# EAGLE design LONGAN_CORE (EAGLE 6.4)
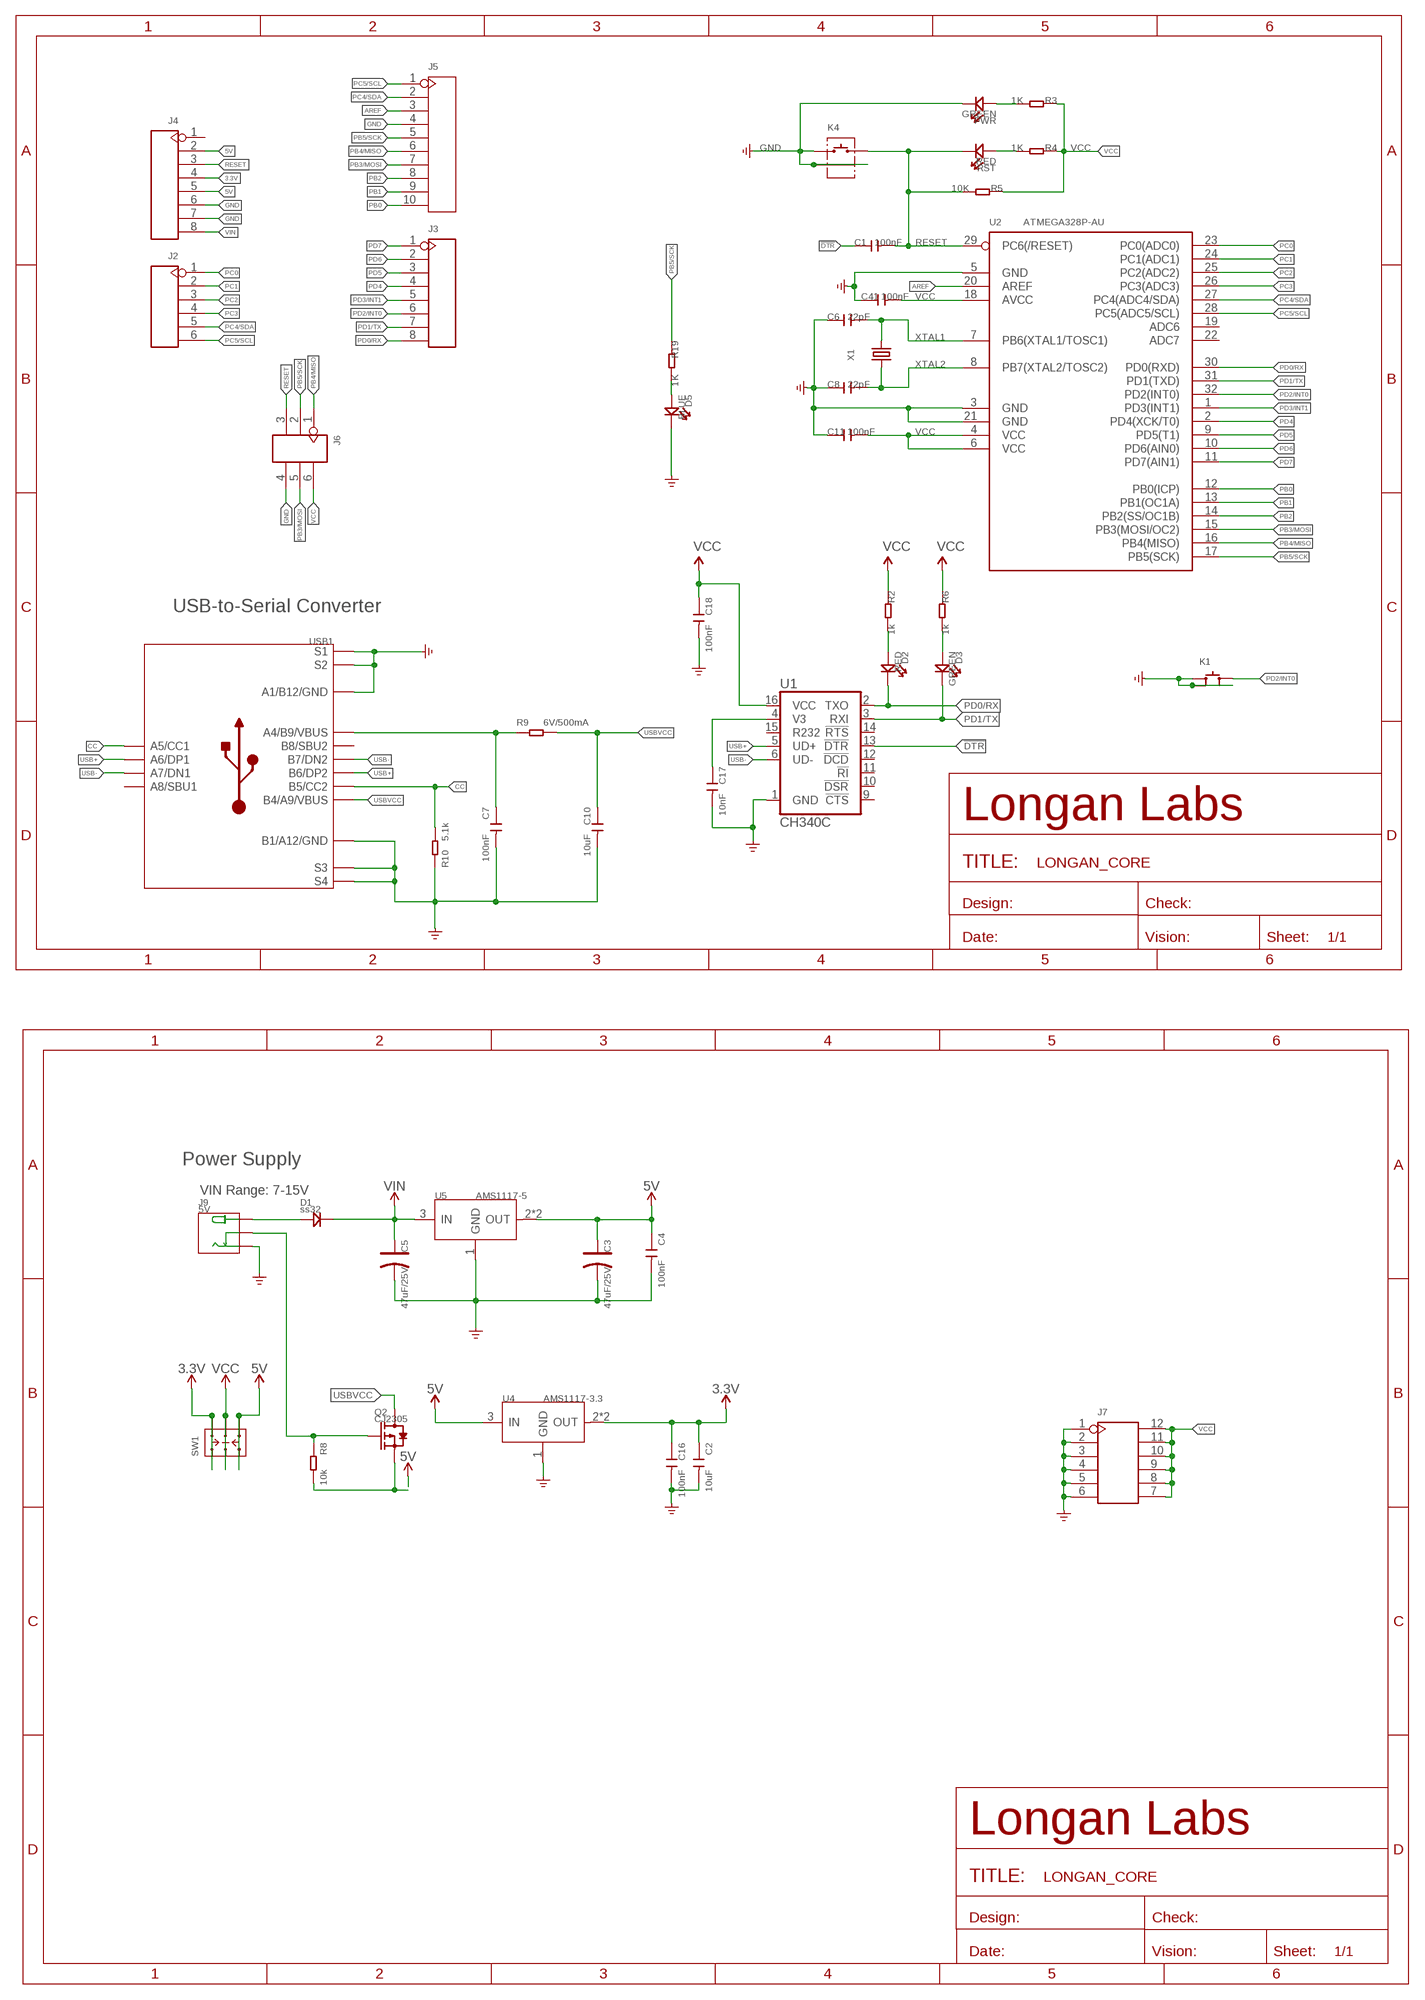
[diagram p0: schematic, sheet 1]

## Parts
C1  100nF  C-0603  [C0603]
C2  10uF  CAP-0603  [C0603]
C3  47uF/25V  CAP-POLAR-ELECTRO-C  [ELECTRO-SMD-C-6MM]
C4  100nF  CAP-0603  [C0603]
C5  47uF/25V  CAP-POLAR-ELECTRO-C  [ELECTRO-SMD-C-6MM]
C6  22pF  C-0603  [C0603]
C7  100nF  CAP-0603  [C0603]
C8  22pF  C-0603  [C0603]
C10  10uF  CAP-0603  [C0603]
C11  100nF  C-0603  [C0603]
C16  100nF  CAP-0603  [C0603]
C17  10nF  CAP-0603  [C0603]
C18  100nF  CAP-0603  [C0603]
C41  100nF  C-0603  [C0603]
D1  ss32  DIODE'SMA'  [DO-214AC]
D2  RED  LED'0603'  [LED-0603]
D3  GREEN  LED'0603'  [LED-0603]
D5  BLUE  LED'0603'  [LED-0603]
J2  HEADER-6P-55/35MIL  [H6-2.54]
J3  HEADER-8P-65/35MIL  [H8-2.54-C65D35MIL]
J4  HEADER-8P-65/35MIL  [H8-2.54-C65D35MIL]
J5  HEADER-10P-2.54  [H10-2.54]
J6  HEADER-2X3P-2.54  [H2X3-2.54]
J7  HEADER-2X6P-2.54  [H2X6-2.54]
J9  5V  POWER-JACK-DC-320120003  [DCJ3P-14.2X11.0X9.0MM]
K1  BUTTON-4P-6.2X6.2  [SW4-SMD-6.2X6.2MM]
K4  BUTTON-2+2P  [SW2+2P-7.7X2.75X3.95MM]
PWR  GREEN  LED'0603'  [LED-0603]
Q2  CJ2305  MOSFET-P'SI2323CDS/SI2305DS<BR>'  [SOT-23]
R2  1k  R-0603  [R0603]
R3  1K  R-0603  [R0603]
R4  1K  R-0603  [R0603]
R5  10K  R-0603  [R0603]
R6  1k  R-0603  [R0603]
R8  10k  RES-0603  [R0603]
R9  6V/500mA  RES-0805  [R0805]
R10  5.1k  RES-0603  [R0603]
R19  1K  R-0603  [R0603]
RST  RED  LED'0603'  [LED-0603]
SW1  SWITCH-2CH-6P-311010004  [SW6-2.54-9.0X3.5X3.2+2.0MM]
U1  CH340C  [SO016]
U2  ATMEGA328P-AU  MCU-ATMEGA8/168/328'AU'  [TQFP32-0.8-7X7MM]
U4  AMS1117-3.3  PMIC-CJ1117S  [SOT-223]
U5  AMS1117-5  PMIC-CJ1117S  [SOT-223]
USB1  TYPE-C-31-M-12  USB2.0-TYPE-C  [USB2.0-TYPE-C]
X1  16MHz  CRYSTAL-2P'HC49US'  [HC49US]

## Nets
3.3V: C2.1 C16.1 J4.4 SW1.CH1A SW1.CH2A U4.2(OUT) U4.TER(OUT)
5V: C3.+ C4.1 J4.2 J4.5 Q2.2(S) R8.2 SW1.CH1B SW1.CH2B U4.3(IN) U5.2(OUT) U5.TER(OUT)
!DTR: C1.1 U1.13(!DTR)
AREF: J5.3 U2.20(AREF)
CC: R10.2 USB1.A5(A5/CC1) USB1.B5(B5/CC2)
GND: C2.2 C3.- C4.2 C5.- C6.1 C7.2 C8.1 C10.2 C11.1 C16.2 C17.2 C18.2 C41.1 D5.- J4.6 J4.7 J5.4 J6.4 J7.1 J7.2 J7.3 J7.4 J7.5 J7.6 J9.-1(-) K1.1(A0) K1.3(B1) K1.4(A1) K4.1 K4.S1 K4.S2 PWR.- R10.1 U1.1(GND) U2.3(GND) U2.5(GND) U2.21(GND) U4.1(GND) U5.1(GND) USB1.A1_B12(A1/B12/GND) USB1.B1_A12(B1/A12/GND) USB1.S1 USB1.S2 USB1.S3 USB1.S4 USB1.S5(S1) USB1.S6(S2) ; supply symbol labelled GND_POWER
INSERT: J9.-2(CDN) Q2.1(G) R8.1
N$3: D5.+ R19.2
N$4: C7.1 R9.1 USB1.A4_B9(A4/B9/VBUS)
N$5: D3.+ R6.2
N$6: C17.1 U1.4(V3)
N$7: PWR.+ R3.2
N$9: D2.+ R2.2
N$17: R4.2 RST.+
PB0: J5.10 U2.12(PB0(ICP))
PB1: J5.9 U2.13(PB1(OC1A))
PB2: J5.8 U2.14(PB2(SS/OC1B))
PB3/MOSI: J5.7 J6.5 U2.15(PB3(MOSI/OC2))
PB4/MISO: J5.6 J6.1 U2.16(PB4(MISO))
PB5/SCK: J5.5 J6.2 R19.1 U2.17(PB5(SCK))
PC0: J2.1 U2.23(PC0(ADC0))
PC1: J2.2 U2.24(PC1(ADC1))
PC2: J2.3 U2.25(PC2(ADC2))
PC3: J2.4 U2.26(PC3(ADC3))
PC4/SDA: J2.5 J5.2 U2.27(PC4(ADC4/SDA))
PC5/SCL: J2.6 J5.1 U2.28(PC5(ADC5/SCL))
PD0/RX: D2.- J3.8 U1.2(TXO) U2.30(PD0(RXD))
PD1/TX: D3.- J3.7 U1.3(RXI) U2.31(PD1(TXD))
PD2/INT0: J3.6 K1.2(B0) U2.32(PD2(INT0))
PD3/INT1: J3.5 U2.1(PD3(INT1))
PD4: J3.4 U2.2(PD4(XCK/T0))
PD5: J3.3 U2.9(PD5(T1))
PD6: J3.2 U2.10(PD6(AIN0))
PD7: J3.1 U2.11(PD7(AIN1))
PWRIN: D1.1(+) J9.+
RESET: C1.2 J4.3 J6.3 K4.2 R5.2 RST.- U2.29(PC6(/RESET))
USB+: U1.5(UD+) USB1.A6(A6/DP1) USB1.B6(B6/DP2)
USB-: U1.6(UD-) USB1.A7(A7/DN1) USB1.B7(B7/DN2)
USBVCC: C10.1 Q2.3(D) R9.2 USB1.B4_A9(B4/A9/VBUS)
VCC: C11.2 C18.1 C41.2 J6.6 J7.7 J7.8 J7.9 J7.10 J7.11 J7.12 R2.1 R3.1 R4.1 R5.1 R6.1 SW1.COM1 SW1.COM2 U1.16(VCC) U2.4(VCC) U2.6(VCC) U2.18(AVCC)
VIN: C5.+ D1.2(-) J4.8 U5.3(IN)
XTAL1: C6.2 U2.7(PB6(XTAL1/TOSC1)) X1.2
XTAL2: C8.2 U2.8(PB7(XTAL2/TOSC2)) X1.1
Unconnected: J4.1 U1.9(!CTS) U1.10(!DSR) U1.11(!RI) U1.12(!DCD) U1.14(!RTS) U1.15(R232) U2.19(ADC6) U2.22(ADC7) USB1.A8(A8/SBU1) USB1.B8(B8/SBU2)

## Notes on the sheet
- USB-to-Serial Converter
- Power Supply
- VIN Range: 7-15V

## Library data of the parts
C1 C6 C8 C11 C41 = Discrete:C*: Ceramic Capacitors
C2 C4 C7 C10 C16-C18 = Discrete-new:CAP: Ceramic Capacitors
C3 C5 = Discrete-new:CAP-POLAR: Electrolytic Capacitors,Tantalum Capacitors and Super Capacitors
D1 = Discrete-new:DIODE
D2 D3 D5 PWR RST = Discrete-new:LED
J2 = Connector-new:HEADER-6P
J3 J4 = Connector-new:HEADER-8P
J5 = Connector-new:HEADER-10P
J6 = Connector-new:HEADER-2X3P
J7 = Connector-new:HEADER-2X6P
J9 = Connector-new:POWER-JACK-DC
K1 = Switch:BUTTON-4P
K4 = Connector-new:BUTTON-2+2P
Q2 = Discrete-new:MOSFET-P
R2-R6 R19 = Discrete:R*
R8-R10 = Discrete-new:RES
SW1 = Switch:SWITCH-2CH-6P
U1 = SparkFun-IC-Comms:CH340C; PROD_ID: IC-14038
U2 = IC-new:MCU-ATMEGA8/168/328
U4 U5 = IC-new:PMIC-CJ*1117: Low Drop Fixed And Adjustable Positive Voltage Regulators http://www.datasheetcatalog.org/datasheet/SGSThomsonMicroelectronics/mXuqtqv.pdf
USB1 = Connector-new:USB2.0-TYPE-C
X1 = Discrete-new:CRYSTAL-2P

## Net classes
1 power: width 0.152 mm, drill 0.152 mm, clearance 0.152 mm
2 gnd: width 0.152 mm, drill 0.152 mm, clearance 0.152 mm
3 usbvcc: width 0.152 mm, drill 0.152 mm, clearance 0.152 mm

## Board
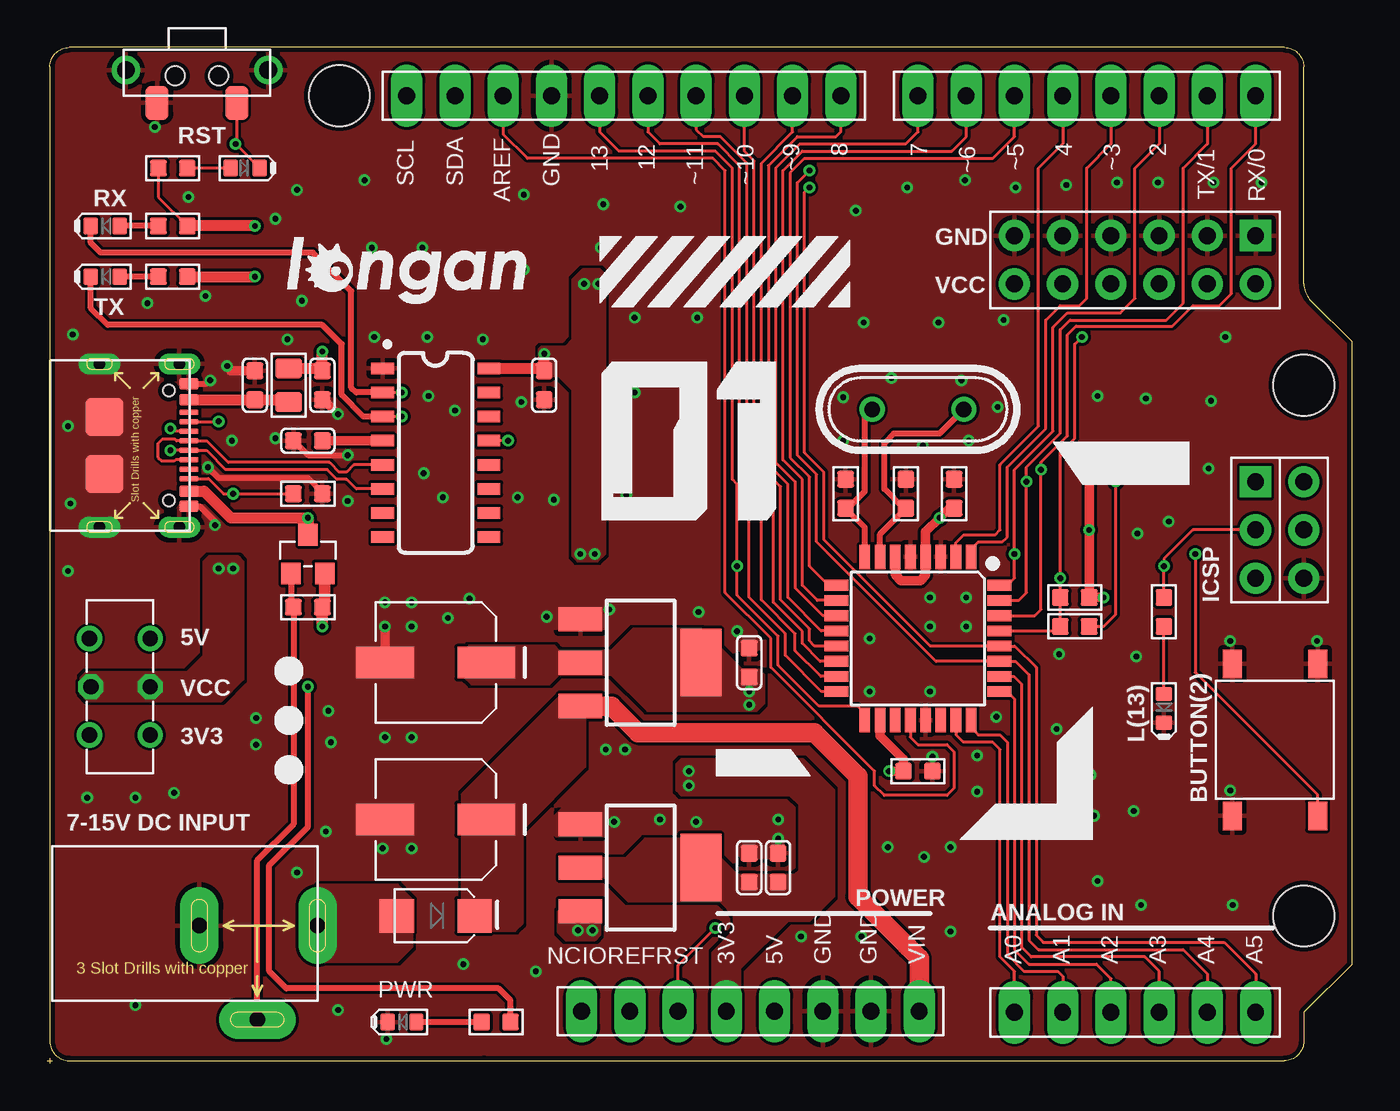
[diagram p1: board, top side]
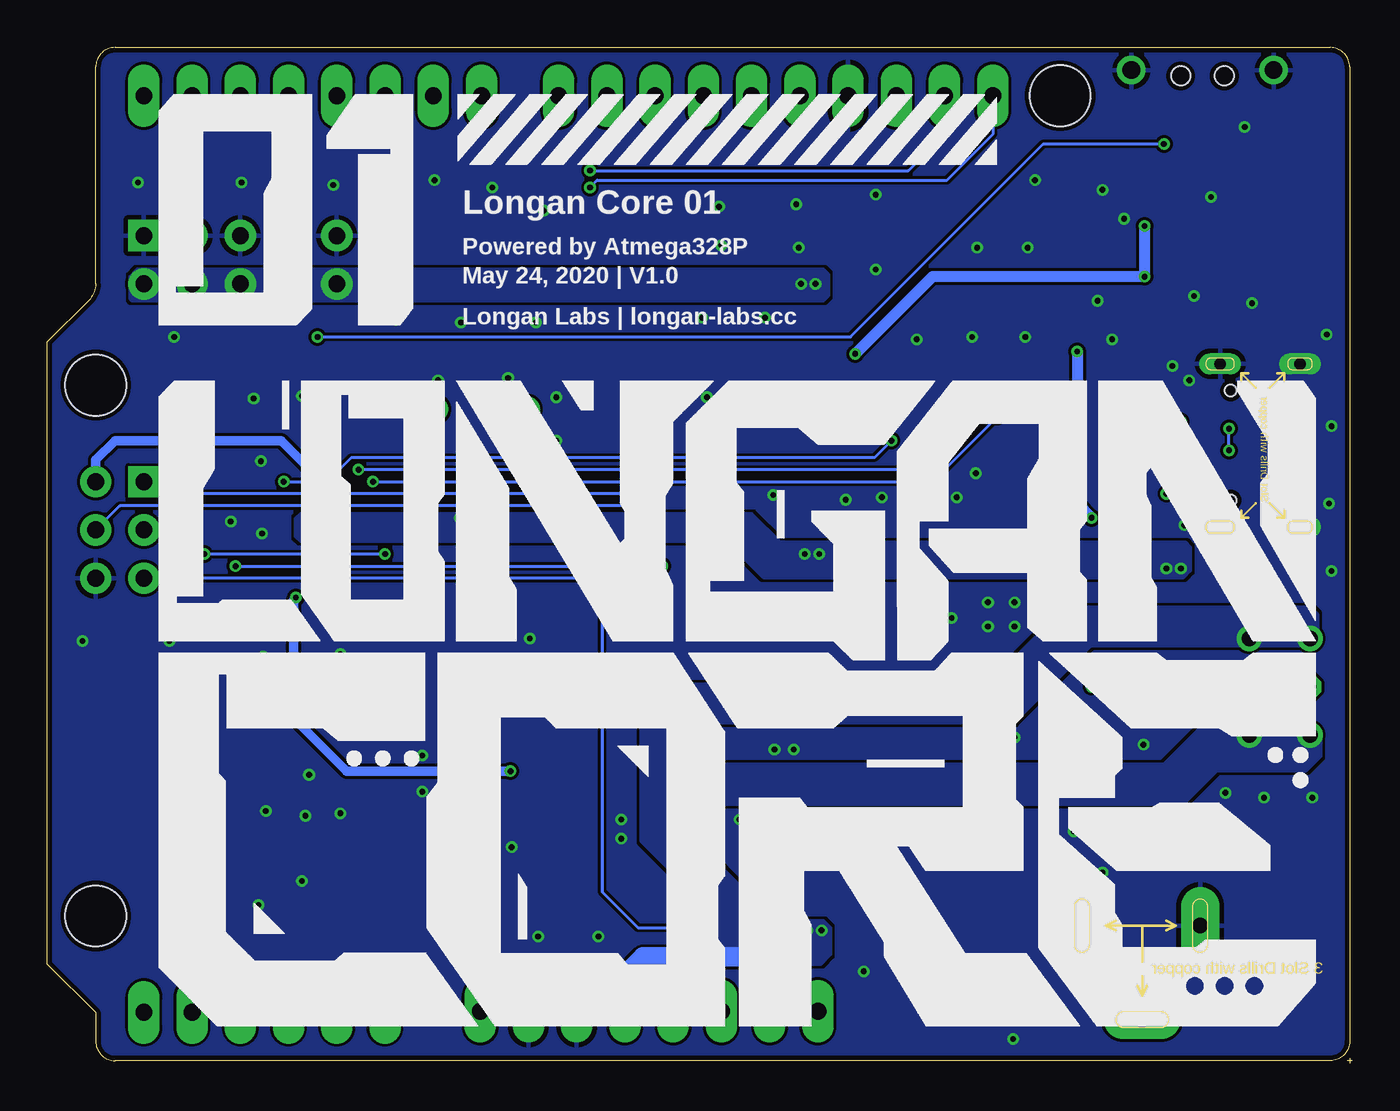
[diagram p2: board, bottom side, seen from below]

Size 68.71 x 53.47 mm. Coordinates in mm from the lower left corner, seen from the top.
Outline: 66.17,41.04 arc45 66.54,40.14 68.71,37.97 68.71,5.21 66.17,2.67 66.17,1.14 arc-90 65.15,0.13 23,0.13
Outline: 66.17,41.02 66.17,52.45 arc90 65.15,53.47 1.14,53.47 arc90 0.13,52.45 0.13,1.14 arc90 1.14,0.13 22.98,0.13
Outline: 0,0.13 0.13,0.13
Outline: 0.13,0.13 0.25,0.13
Outline: 0.13,0.25 0.13,0.13
Outline: 0.13,0.13 0.13,0
Copper layers (1*16): Top 0.035mm / dielectric 1.5mm / Bottom 0.035mm
Design rules "SeeedStudio_2layer_DRU_no_angle_20140221 *": minimum track width 6mil, minimum drill 10mil, track to track 6mil, track to pad 6mil, pad to pad 6mil, via to via 6mil, smd to smd 0mil, copper to edge 10mil, drill to drill 10mil, minimum pad ring 10mil, minimum via ring 6mil, stop-mask expansion 2mil, vias tented up to drill 100mil, thermal gap 10mil
Holes 3.2 mm at 15.37,50.93 66.17,35.69 66.17,7.75

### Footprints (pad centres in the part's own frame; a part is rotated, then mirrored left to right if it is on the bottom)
C0603 = smd 0.889 x 0.889: 1 -0.762,0; 2 0.762,0
ELECTRO-SMD-C-6MM = smd 3.048 x 1.651: + 2.667,0; - -2.667,0
DO-214AC = smd 1.8 x 1.77: 1 2.042,0; 2 -2.042,0
LED-0603 = smd 0.762 x 0.889: + 0.762,0; - -0.762,0
H6-2.54 = drill 0.889 pad 1.651 long: 1 0,6.35; 2 0,3.81; 3 0,1.27; 4 0,-1.27; 5 0,-3.81; 6 0,-6.35
H8-2.54-C65D35MIL = drill 0.889 pad 1.651 long: 1 0,8.89; 2 0,6.35; 3 0,3.81; 4 0,1.27; 5 0,-1.27; 6 0,-3.81; 7 0,-6.35; 8 0,-8.89
H10-2.54 = drill 0.889 pad 1.651 long: 1 0,11.43; 2 0,8.89; 3 0,6.35; 4 0,3.81; 5 0,1.27; 6 0,-1.27; 7 0,-3.81; 8 0,-6.35; 9 0,-8.89; 10 0,-11.43
H2X3-2.54 = drill 0.889 pad 1.651 square: 1 -1.27,2.54 | drill 0.889 pad 1.651: 2 -1.27,0; 3 -1.27,-2.54; 4 1.27,-2.54; 5 1.27,0; 6 1.27,2.54
H2X6-2.54 = drill 0.889 pad 1.651 square: 1 -1.27,6.35 | drill 0.889 pad 1.651: 2 -1.27,3.81; 3 -1.27,1.27; 4 -1.27,-1.27; 5 -1.27,-3.81; 6 -1.27,-6.35; 7 1.27,-6.35; 8 1.27,-3.81; 9 1.27,-1.27; 10 1.27,1.27; 11 1.27,3.81; 12 1.27,6.35
DCJ3P-14.2X11.0X9.0MM = drill 0.813 pad 2.032 long: + 3.175,0; -1 -3.048,0; -2 0,-4.953
SW4-SMD-6.2X6.2MM = smd 1.5 x 1: 1 -4,2.25; 2 -4,-2.25; 3 4,-2.25; 4 4,2.25
SW2+2P-7.7X2.75X3.95MM = smd 1.2 x 1.778: 1 -2.1,-0.127; 2 2.1,-0.127 | drill 0.924 pad 1.5: S1 -3.75,1.6; S2 3.75,1.6 | hole 1: -1.15,1.3; 1.15,1.3
SOT-23 = smd 1.143 x 1.016: 1 1.016,-0.889; 2 1.016,0.889; 3 -1.016,0
R0603 = smd 0.889 x 0.889: 1 -0.762,0; 2 0.762,0
R0805 = smd 1.016 x 1.397: 1 -0.889,0; 2 0.889,0
SW6-2.54-9.0X3.5X3.2+2.0MM = drill 0.813 pad 1.27: CH1A -2.54,-1.6; CH1B 2.54,-1.6; CH2A -2.54,1.6; CH2B 2.54,1.6 | drill 0.813 pad 1.27 octagon: COM1 0,-1.6; COM2 0,1.524
SO016 = smd 0.6 x 1.2: 1 -4.445,-2.8; 2 -3.175,-2.8; 3 -1.905,-2.8; 4 -0.635,-2.8; 5 0.635,-2.8; 6 1.905,-2.8; 7 3.175,-2.8; 8 4.445,-2.8; 9 4.445,2.8; 10 3.175,2.8; 11 1.905,2.8; 12 0.635,2.8; 13 -0.635,2.8; 14 -1.905,2.8; 15 -3.175,2.8; 16 -4.445,2.8
TQFP32-0.8-7X7MM = smd 1.27 x 0.559: 1 -4.293,2.8; 2 -4.293,2; 3 -4.293,1.2; 4 -4.293,0.4; 5 -4.293,-0.4; 6 -4.293,-1.2; 7 -4.293,-2; 8 -4.293,-2.8; 17 4.293,-2.8; 18 4.293,-2; 19 4.293,-1.2; 20 4.293,-0.4; 21 4.293,0.4; 22 4.293,1.2; 23 4.293,2; 24 4.293,2.8 | smd 0.559 x 1.27: 9 -2.8,-4.293; 10 -2,-4.293; 11 -1.2,-4.293; 12 -0.4,-4.293; 13 0.4,-4.293; 14 1.2,-4.293; 15 2,-4.293; 16 2.8,-4.293; 25 2.8,4.293; 26 2,4.293; 27 1.2,4.293; 28 0.4,4.293; 29 -0.4,4.293; 30 -1.2,4.293; 31 -2,4.293; 32 -2.8,4.293
SOT-223 = smd 1.27 x 2.286: 1 -2.286,-3.175; 2 0,-3.175; 3 2.286,-3.175 | smd 3.556 x 2.159: TER 0,3.175
USB2.0-TYPE-C = smd 1 x 0.6: A1_B12 -0.05,3.25; A4_B9 -0.05,2.4; B1_A12 -0.05,-3.2; B4_A9 -0.05,-2.4 | smd 1 x 0.3: A5 -0.05,1.25; A6 -0.05,0.25; A7 -0.05,-0.25; A8 -0.05,-1.25; B5 -0.05,-1.75; B6 -0.05,-0.75; B7 -0.05,0.75; B8 -0.05,1.75 | drill 0.6 pad 1 long: S1 -4.75,4.3; S2 -4.75,-4.3 | drill 0.6 pad 1.1 long: S3 -0.55,4.3; S4 -0.55,-4.3 | smd 2 x 2: S5 -4.5,1.5; S6 -4.5,-1.5 | hole 0.6: -1.1,-2.89; -1.1,2.89
HC49US = drill 0.813: 1 -2.413,0; 2 2.413,0

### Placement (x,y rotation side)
C1  54.1,22.99 180 top
C2  36.96,10.29 90 top
C3  20.45,21.08 0 top
C4  36.96,21.08 90 top
C5  20.45,12.83 0 top
C6  45.21,29.97 270 top
C7  10.92,35.69 90 top
C8  42.04,29.97 270 top
C10  14.48,35.69 270 top
C11  47.75,29.97 270 top
C16  38.48,10.29 90 top
C17  13.72,32.77 180 top
C18  26.16,35.69 270 top
C41  45.85,15.37 180 top
D1  20.45,7.75 180 top
D2  3.05,44.07 0 top
D3  3.05,41.4 0 top
D5  58.8,18.67 90 top
J2  57.28,2.67 90 top
J3  54.74,50.93 90 top
J4  37.02,2.73 90 top
J5  30.35,50.93 90 top
J6  64.9,28.07 0 top
J7  57.28,42.29 270 top
J9  11.05,7.24 0 top
K1  64.64,17.02 90 top
K4  7.87,50.67 0 top
PWR  18.67,2.16 0 top
Q2  13.72,26.8 270 top
R2  6.6,44.07 180 top
R3  23.62,2.16 180 top
R4  6.6,47.12 0 top
R5  54.1,24.51 180 top
R6  6.6,41.4 180 top
R8  13.72,24 0 top
R9  12.7,35.69 90 top
R10  13.72,29.97 180 top
R19  58.8,23.75 270 top
RST  10.41,47.12 180 top
SW1  3.81,19.81 90 top
U1  20.45,32.13 270 top
U2  45.85,22.35 270 top
U4  31.24,10.29 270 top
U5  31.24,21.08 270 top
USB1  7.49,32.51 0 top
X1  45.85,34.42 0 top

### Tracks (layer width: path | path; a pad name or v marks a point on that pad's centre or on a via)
3.3V  (via drill 0.3 pad 0.61)
  other vias: 33.78,15.37 33.78,14.61
  pour Top (isolate 0.254, no thermals): 27.81,10.79 30.48,10.79 31.5,11.81 34.42,11.81 36.32,9.91 39.37,9.91 39.62,10.16 39.62,13.59 39.12,14.1 33.4,14.1 33.15,14.35 33.15,15.75 33.4,16 39.79,16 41.4,14.39 41.4,8.76 40.13,7.49 38.99,7.49 36.45,4.95 36.45,1.91 36.07,1.52 35.43,1.52 35.05,1.91 35.05,5.84 36.2,6.98 36.2,7.75 35.43,8.51 30.61,8.51 29.34,9.78 27.69,9.78 27.56,9.91 27.56,10.54
  pour Bottom (isolate 0.254, no thermals): 33.78,15.75 9.91,15.75 7.75,17.91 2.16,17.91 1.65,17.4 1.65,16.13 2.41,15.37 7.11,15.37 8.89,13.59 33.78,13.59 34.29,14.1 34.29,15.37 33.91,15.75
5V  (via drill 0.3 pad 0.61)
  Top 0.61: v14.48,22.99 R8.2 14.61,24.13 Q2.2
  Bottom 1.016: J4.5 38.29,4.63 37.34,5.59 30.99,5.59
  other vias: 36.96,19.56 36.96,18.86 28.7,6.98 27.94,6.98
  pour Top (isolate 0.254, no thermals): 22.22,21.97 26.67,21.97 26.92,21.72 29.72,21.72 30.86,22.86 34.42,22.86 36.58,20.7 37.47,20.7 37.72,20.45 37.72,18.92 37.34,18.54 31.62,18.54 29.72,20.45 26.92,20.45 26.42,19.94 22.35,19.94 21.97,20.32 21.97,21.72
  pour Bottom (isolate 0.254, no thermals): 35.69,12.83 35.69,16.94 34.72,17.91 17.78,17.91 13.72,21.97 2.03,21.97 1.78,22.22 1.78,23.62 2.16,24 15.11,24 19.18,19.94 37.08,19.94 37.47,19.56 37.47,11.68 33.78,8 33.78,5.97 33.53,5.71 31.5,5.71 31.37,5.59 31.37,2.41 30.99,2.03 30.1,2.03 29.97,2.16 29.97,4.44 29.21,5.21 27.94,5.21 27.43,5.71 27.43,7.11 27.81,7.49 30.35,7.49
  pour Top (isolate 0.254, no thermals): 27.81,8.38 28.7,8.38 29.08,8 29.08,6.73 28.83,6.48 27.3,6.48 26.92,6.86 26.92,8 27.3,8.38
!DTR  (via drill 0.3 pad 0.61)
  Top 0.152: C1.1 55.63,22.99 56.26,23.62 v56.26,30.61 | v24.26,32.77 U1.13
  Bottom 0.152: v24.26,32.77 25.15,31.88 52.71,31.88 53.98,30.61 v56.26,30.61
AREF
  Top 0.152: U2.20 45.45,17.16 45.85,16.76 47.37,16.76 47.75,16.38 47.75,14.48 47.37,14.1 44.07,14.1 43.56,14.61 43.56,15.37 38.1,20.83 38.1,22.35 35.69,24.77 35.69,46.99 35.05,47.62 25.27,47.62 24,48.9 J5.3
CC  (via drill 0.3 pad 0.61)
  Top 0.152: USB1.B5 8.48,30.76 9.27,29.97 9.65,29.97 v9.78,29.97 R10.2 | USB1.A5 9,33.76 v9.02,33.78
  Bottom 0.152: v9.02,33.78 9.02,30.73 v9.78,29.97
GND  (via drill 0.3 pad 0.61)
  Top 0.305: R10.1 14.48,30.04 13.72,30.8 9.02,30.8 v8.45,31.37 | C17.2 13.72,32 v15.81,32 | USB1.B1_A12 8.03,29.31 8.89,28.45 8.89,28.38 v8.83,28.32 | USB1.A1_B12 8.33,35.76 8.51,35.94 v8.57,35.94
  Top 0.508: C3.- v17.78,22.99 | C7.2 9.65,36.45 9.4,36.7 v9.46,36.7 | C10.2 14.54,34.93 v15.3,34.16
  other vias: 19.18,22.99 19.18,24.26 17.78,24.26 17.78,17.14 19.18,17.14 19.18,11.3 17.65,11.3 29.59,23.88 26.29,23.49 34.29,23.75 36.32,22.73 29.84,12.7 32.26,12.83 34.16,12.7 38.48,12.83 38.48,11.81 17.84,1.27 46.61,16.13 46.48,19.56 43.31,19.56 43.31,22.35 46.48,22.99 48.39,22.99 48.39,24.51 46.48,24.51 48.51,32.77 41.91,32.77 41.91,35.05 44.45,36.07 48.13,35.94 50.04,34.54 46.1,32.51 57.47,31.69 61.15,31.31 61.28,34.86 57.85,34.99 55.12,13.02 62.29,14.35 62.29,22.22 66.87,22.22 39.69,6.67 42.86,6.67 47.56,6.92 47.56,11.37 44.26,11.37 46.16,10.86 55.31,9.59 53.28,13.14 53.15,17.59 53.28,21.53 57.34,21.4 54.93,15.18 57.21,13.27 57.59,8.32 62.42,8.32 62.04,38.23 63.94,46.36 61.4,46.36 58.48,46.36 56.32,46.36 53.66,46.23 50.99,46.1 48.32,46.48 45.28,46.1 42.57,44.88 42.99,38.99 46.93,38.99 50.36,39.12 34.23,39.24 30.92,39.24 30.92,35.31 33.97,35.05 24.96,34.8 22.92,38.1 25.08,41.78 25.08,45.72 29.27,45.21 33.21,43.05 29.15,42.93 33.34,45.09 20,38.23 17.21,38.23 17.08,42.93 19.75,42.93 16.7,46.48 13.14,45.97 12,44.45 13.4,40.13 8.32,40.39 5.27,40.01 7.43,45.59 12.64,38.1 12,32.89 15.81,29.59 9.72,32.77 5.65,49.28 1.33,38.35 1.08,33.53 1.21,29.46 1.08,25.91 10.99,18.16 10.99,16.76 14.92,16.89 14.8,18.54 14.67,12.19 13.14,10.03 6.67,14.22 4.64,13.97 2.1,13.97 15.3,2.79 4.64,3.05 21.91,5.21 25.72,4.83 29.4,16.51 30.42,16.51 30.48,29.91 33.66,29.78 26.67,29.65 24.77,29.78 20.83,29.78 19.81,31.05 20.07,35.12 21.46,34.35 22.22,24.45 21.08,23.43 48.96,14.29 48.96,16.19 49.97,18.22 55.31,35.12 57.4,27.88 59.05,28.51
  pour Top (isolate 0.152, rank 6): 0.13,53.47 68.71,53.47 68.71,0.13 0.13,0.13
  pour Bottom (isolate 0.152, rank 6): 0.13,53.47 68.71,53.47 68.71,0.13 2.67,0.13 2.67,-0.51 0.13,-0.51
  pour Top (isolate 0.254, no thermals): 17.65,24.64 16.64,24.64 16,24 16,11.43 16.76,10.67 19.43,10.67 19.81,11.05 19.81,24.26 19.43,24.64
  pour Top (isolate 0.254, no thermals): 36.07,22.22 36.07,22.99 35.69,23.37 29.84,23.37 29.34,22.86 25.15,22.86 24.89,23.11 24.89,24.77 25.27,25.15 34.93,25.15 37.47,22.61 37.47,21.84 37.21,21.59 36.58,21.59 36.07,22.1
  pour Top (isolate 0.254, no thermals): 29.59,13.46 38.23,13.46 38.73,12.95 38.73,10.92 38.61,10.79 36.58,10.79 36.32,11.05 36.32,12.07 35.94,12.45 30.35,12.45 29.84,11.94 26.8,11.94 26.67,12.07 26.67,12.95 27.18,13.46
INSERT
  Top 0.305: Q2.1 12.83,24.13 R8.1 12.95,12.57 11.05,10.67 J9.-2
N$3
  Top 0.152: D5.+ R19.2
N$4
  Top 0.584: USB1.A4_B9 10.91,34.91 C7.1 12.57,34.93 R9.1
N$5
  Top 0.305: R6.2 D3.+
N$6
  Top 0.508: C17.1 U1.4
N$7
  Top 0.305: R3.2 PWR.+
N$9
  Top 0.305: R2.2 D2.+
N$17
  Top 0.152: RST.+ R4.2
PB0
  Top 0.152: U2.12 40.75,22.75 38.99,24.51 38.99,30.48 38.86,30.61 38.8,30.67 37.97,31.5 37.97,47.24 39.5,48.77 41.53,48.77 41.78,49.02 J5.10
PB1
  Top 0.152: U2.13 40.41,21.95 40.13,22.22 40.13,22.86 38.61,24.38 38.61,30.35 37.59,31.37 37.59,47.37 39.24,49.02 J5.9
PB2
  Top 0.152: U2.14 40.7,21.15 39.75,22.1 39.75,22.73 38.23,24.26 38.23,30.23 37.21,31.24 37.21,47.5 36.77,47.94 36.7,48.01 J5.8
PB3/MOSI  (via drill 0.3 pad 0.61)
  Top 0.152: U2.15 40.73,20.35 39.37,21.72 39.37,22.61 37.59,24.38 v37.59,29.34 37.59,30.35 36.83,31.11 36.83,47.37 35.43,48.77 34.54,48.77 34.16,49.15 J5.7
  Bottom 0.152: v37.59,29.34 64.9,29.34 J6.5
PB4/MISO  (via drill 0.3 pad 0.61)
  Top 0.152: U2.16 40.77,19.55 38.86,21.46 38.86,22.61 36.96,24.51 v36.96,29.97 36.96,30.48 36.45,30.99 36.45,47.24 35.31,48.39 32.26,48.39 31.62,49.02 J5.6
  Bottom 0.152: v36.96,29.97 62.99,29.97 J6.1
PB5/SCK  (via drill 0.3 pad 0.61)
  Top 0.152: U2.17 43.05,18.42 42.67,18.8 40.64,18.8 38.48,20.95 38.48,22.48 36.32,24.64 v36.32,26.16 36.32,30.48 36.07,30.73 36.07,47.12 35.18,48.01 30.1,48.01 29.08,49.02 J5.5 | R19.1 v58.8,26.16 58.8,26.54 60.33,28.07 J6.2
  Bottom 0.152: v58.8,26.16 v36.32,26.16
PC0
  Top 0.152: U2.23 47.85,17.27 48.23,16.89 49.78,16.89 50.16,16.51 50.16,5.59 50.93,4.83 J2.1
PC1
  Top 0.152: U2.24 48.65,17.65 49.02,17.27 50.16,17.27 50.55,16.89 50.55,5.71 51.44,4.83 53.21,4.83 53.47,4.57 J2.2
PC2
  Top 0.152: U2.25 50.55,19.55 50.93,19.18 50.93,5.97 51.69,5.21 55.25,5.21 56.01,4.44 J2.3
PC3
  Top 0.152: U2.26 50.9,20.35 51.31,19.94 51.31,6.1 51.82,5.59 57.79,5.59 58.55,4.83 J2.4
PC4/SDA  (via drill 0.3 pad 0.61)
  Top 0.152: v40.13,46.99 39.5,46.36 39.5,32 40.51,30.99 40.51,27.43 46.79,21.15 U2.27 50.98,21.15 51.69,20.45 51.69,6.48 52.2,5.97 59.82,5.97 61.09,4.7 J2.5
  Bottom 0.152: v40.13,46.99 23.37,46.99 21.72,48.64 21.59,48.77 21.46,48.9 J5.2
PC5/SCL  (via drill 0.3 pad 0.61)
  Top 0.152: v40.13,46.1 39.88,45.85 39.88,32.13 40.89,31.11 40.89,27.56 46.5,21.95 U2.28 50.95,21.95 52.07,20.83 52.07,6.73 52.45,6.35 61.98,6.35 63.63,4.7 J2.6
  Bottom 0.152: v40.13,46.1 39.75,46.48 21.34,46.48 18.92,48.9 J5.1
PD0/RX  (via drill 0.3 pad 0.61)
  Top 0.152: U2.30 52,23.55 52.32,23.88 v52.32,31.24 52.32,31.62 53.72,33.02 53.72,38.35 54.16,38.8 59.25,38.8 60.33,39.88 61.72,39.88 62.36,40.51 62.36,47.12 63.63,48.39 J3.8 | U1.2 v18.67,35.31
  Top 0.305: U1.2 16.26,35.31 16,35.56 16,40.64 13.97,42.67 2.79,42.67 2.29,43.18 D2.-
  Bottom 0.152: v18.67,35.31 18.67,34.93 22.35,31.24 v52.32,31.24
PD1/TX  (via drill 0.3 pad 0.61)
  Top 0.152: U2.31 51.15,24.35 51.56,24.77 v51.56,30.61 51.56,31.37 53.34,33.15 53.34,38.61 53.85,39.12 58.93,39.12 59.82,40.01 59.82,47.12 61.09,48.39 J3.7 | v18.67,34.04 U1.3
  Top 0.305: D3.- 2.29,39.75 3.17,38.86 14.48,38.86 15.49,37.85 15.49,35.18 16.64,34.04 U1.3
  Bottom 0.152: v51.56,30.61 22.1,30.61 v18.67,34.04
PD2/INT0  (via drill 0.3 pad 0.61)
  Top 0.152: U2.32 50.55,25.15 50.93,25.53 v50.93,26.8 50.93,31.24 52.96,33.27 52.96,38.73 53.72,39.5 56.52,39.5 57.28,40.26 57.28,47.12 58.55,48.39 J3.6 | v60.45,26.8 60.45,20.57 66.89,14.13 K1.2
  Bottom 0.152: v50.93,26.8 v60.45,26.8
PD3/INT1
  Top 0.152: U2.1 48.65,27.06 49.02,27.43 50.29,27.43 50.55,27.69 50.55,31.37 52.58,33.4 52.58,39.12 53.34,39.88 54.36,39.88 54.74,40.26 54.74,47.12 56.01,48.39 J3.5
PD4
  Top 0.152: U2.2 47.85,27.4 48.26,27.81 49.91,27.81 50.16,28.07 50.16,31.5 52.2,33.53 52.2,47.12 53.47,48.39 J3.4
PD5
  Top 0.152: U2.9 41.14,25.15 40.13,26.16 40.13,30.86 39.12,31.88 39.12,46.86 39.88,47.62 49.78,47.62 50.93,48.77 J3.3
PD6
  Top 0.152: U2.10 40.55,24.35 39.75,25.15 39.75,30.73 38.73,31.75 38.73,46.99 39.75,48.01 47.62,48.01 48.39,48.77 J3.2
PD7
  Top 0.152: U2.11 40.84,23.55 39.37,25.02 39.37,30.61 38.35,31.62 38.35,47.12 39.62,48.39 45.21,48.39 45.85,49.02 J3.1
PWRIN
  pour Top (isolate 0.254, no thermals): 14.48,9.4 18.41,9.4 19.18,8.64 19.18,6.1 18.41,5.33 14.35,5.33 13.46,6.22 13.46,8.51 14.35,9.4
RESET  (via drill 0.3 pad 0.61)
  Top 0.152: U2.29 53.11,22.75 C1.2 R5.2 v53.34,25.53 53.34,32.13 54.1,32.89 54.1,37.85 v54.48,38.23 | K4.2 9.97,48.46 v9.91,48.39 RST.- | J4.3 33.21,5.14 v35.18,7.11
  Bottom 0.152: v54.48,38.23 26.42,38.23 16.26,48.39 v9.91,48.39 | J6.3 v53.34,25.53 40.13,25.53 39.5,24.89 39.5,9.02 37.59,7.11 v35.18,7.11
USB+
  Top 0.152: U1.5 16.13,31.5 15.75,31.11 15.37,31.11 14.86,31.62 9.53,31.62 8.39,32.76 USB1.A6 6.8,32.76 6.73,32.83 6.03,32.83 5.84,32.64 5.84,31.88 6.03,31.69 6.67,31.69 6.74,31.76 USB1.B6
USB-  (via drill 0.3 pad 0.61)
  Top 0.152: U1.6 16.26,30.23 15.75,30.73 15.24,30.73 14.73,31.24 9.4,31.24 8.38,32.26 USB1.A7 v6.48,32.26 | USB1.B7 6.62,33.26 v6.48,33.4
  Bottom 0.152: v6.48,32.26 v6.48,33.4
USBVCC  (via drill 0.3 pad 0.61)
  Top 0.584: R9.2 14.35,36.58 C10.1 v14.48,37.47 | Q2.3 v13.72,28.7 9.65,28.7 8.24,30.11 USB1.B4_A9
  Bottom 0.584: v14.48,37.47 14.48,29.46 v13.72,28.7
VCC  (via drill 0.3 pad 0.61)
  Top 0.152: R4.1 5.84,45.59 R2.1
  Top 0.305: R3.1 24.38,3.3 23.75,3.94 12.57,3.94 11.68,4.83 11.68,10.41 13.72,12.45 v13.72,19.81
  Top 0.508: U2.6 44.65,25.71 44.96,25.4 45.97,25.4 46.25,25.67 U2.4 46.25,27.96 v46.99,28.7 47.5,29.21 C11.2 | v44.32,15.37 C41.2 45.09,16 43.85,17.24 U2.18 | v54.86,31.24 v54.86,28.07 R5.1 v55.63,24.51
  Top 0.584: R6.1 v10.92,41.4 | v10.92,44.07 R2.1 | v26.16,37.34 C18.1 26.04,36.58 U1.16
  Bottom 0.305: SW1.COM1 v13.72,19.81
  Bottom 0.508: J6.6 66.17,31.75 65.15,32.77 56.39,32.77 v54.86,31.24 | v44.32,15.37 52.96,15.37 55.75,18.16 55.75,24.38 v55.63,24.51
  Bottom 0.584: v10.92,44.07 v10.92,41.4 22.1,41.4 v26.16,37.34
  other vias: 9.78,26.04 9.02,26.04 28.07,26.8 28.83,26.8 29.02,41.02 28.26,41.02
  pour Top (isolate 0.254, no thermals): 2.03,20.57 7.37,20.57 8.26,21.46 8.26,26.42 8.51,26.67 10.03,26.67 10.29,26.42 10.29,20.19 9.14,19.05 2.16,19.05 1.78,19.43 1.78,20.32
  pour Bottom (isolate 0.254, no thermals): 8.89,25.53 30.99,25.53 32.89,27.43 55.37,27.43 55.63,27.69 55.63,28.7 55.37,28.96 31.62,28.96 30.1,27.43 8.76,27.43 8.51,27.18 8.51,25.91
  pour Top (isolate 0.254, no thermals): 27.69,26.67 27.69,35.43 26.92,36.2 26.29,36.2 25.91,36.58 25.91,37.59 26.04,37.72 27.3,37.72 27.69,38.1 27.69,41.28 28.19,41.78 29.08,41.78 29.34,41.53 29.34,26.8 28.96,26.42 27.94,26.42
  pour Bottom (isolate 0.254, no thermals): 64.26,40.13 27.81,40.13 27.56,40.39 27.56,41.53 27.81,41.78 64.01,41.78 64.39,41.4 64.39,40.26
VIN
  Top 1.016: U5.3 29.72,18.8 31.11,17.4 40.38,17.4 42.67,15.11 42.67,8.76 45.21,6.22 45.34,6.1 45.91,5.52 J4.8
  pour Top (isolate 0.254, no thermals): 27.81,19.3 26.99,19.3 21.84,14.16 21.84,7.49 22.35,6.98 24.64,6.98 25.02,7.37 25.02,12.32 28.32,15.62 28.32,18.8
XTAL1
  Top 0.305: U2.7 43.85,27.84 C6.2 45.09,29.21 44.07,30.23 44.07,32.64 44.58,33.15 46.99,33.15 X1.2
XTAL2
  Top 0.305: U2.8 43.05,28.2 C8.2 42.16,29.21 43.05,30.1 43.05,34.04 X1.1

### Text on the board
tPlace: RST | 8 | 7 | 4 | 2 | 13 | 12 | ~9 | ~6 | ~5 | ~3 | SCL | SDA | GND | ~11 | ~10 | RX | AREF | TX/1 | RX/0 | GND | VCC | TX | ICSP | 5V | VCC | 3V3 | L(13) | BUTTON(2) | 7-15V DC INPUT | POWER | ANALOG IN | IOREF | RST | NC | 3V3 | 5V | GND | GND | VIN | A0 | A1 | A2 | A3 | A4 | A5 | PWR
bPlace: Longan Core 01 | Powered by Atmega328P | May 24, 2020 | V1.0 | Longan Labs | longan-labs.cc
Modules: USB | Switch | ANALOG | BLE_MODULE

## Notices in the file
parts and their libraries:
SparkFun-Aesthetics: Licensing: CC v3.0 Share-Alike You are welcome to use this library for commercial purposes.
SparkFun-IC-Comms: Licensing: Creative Commons ShareAlike 4.0 International - https://creativecommons.org/licenses/by-sa/4.0
